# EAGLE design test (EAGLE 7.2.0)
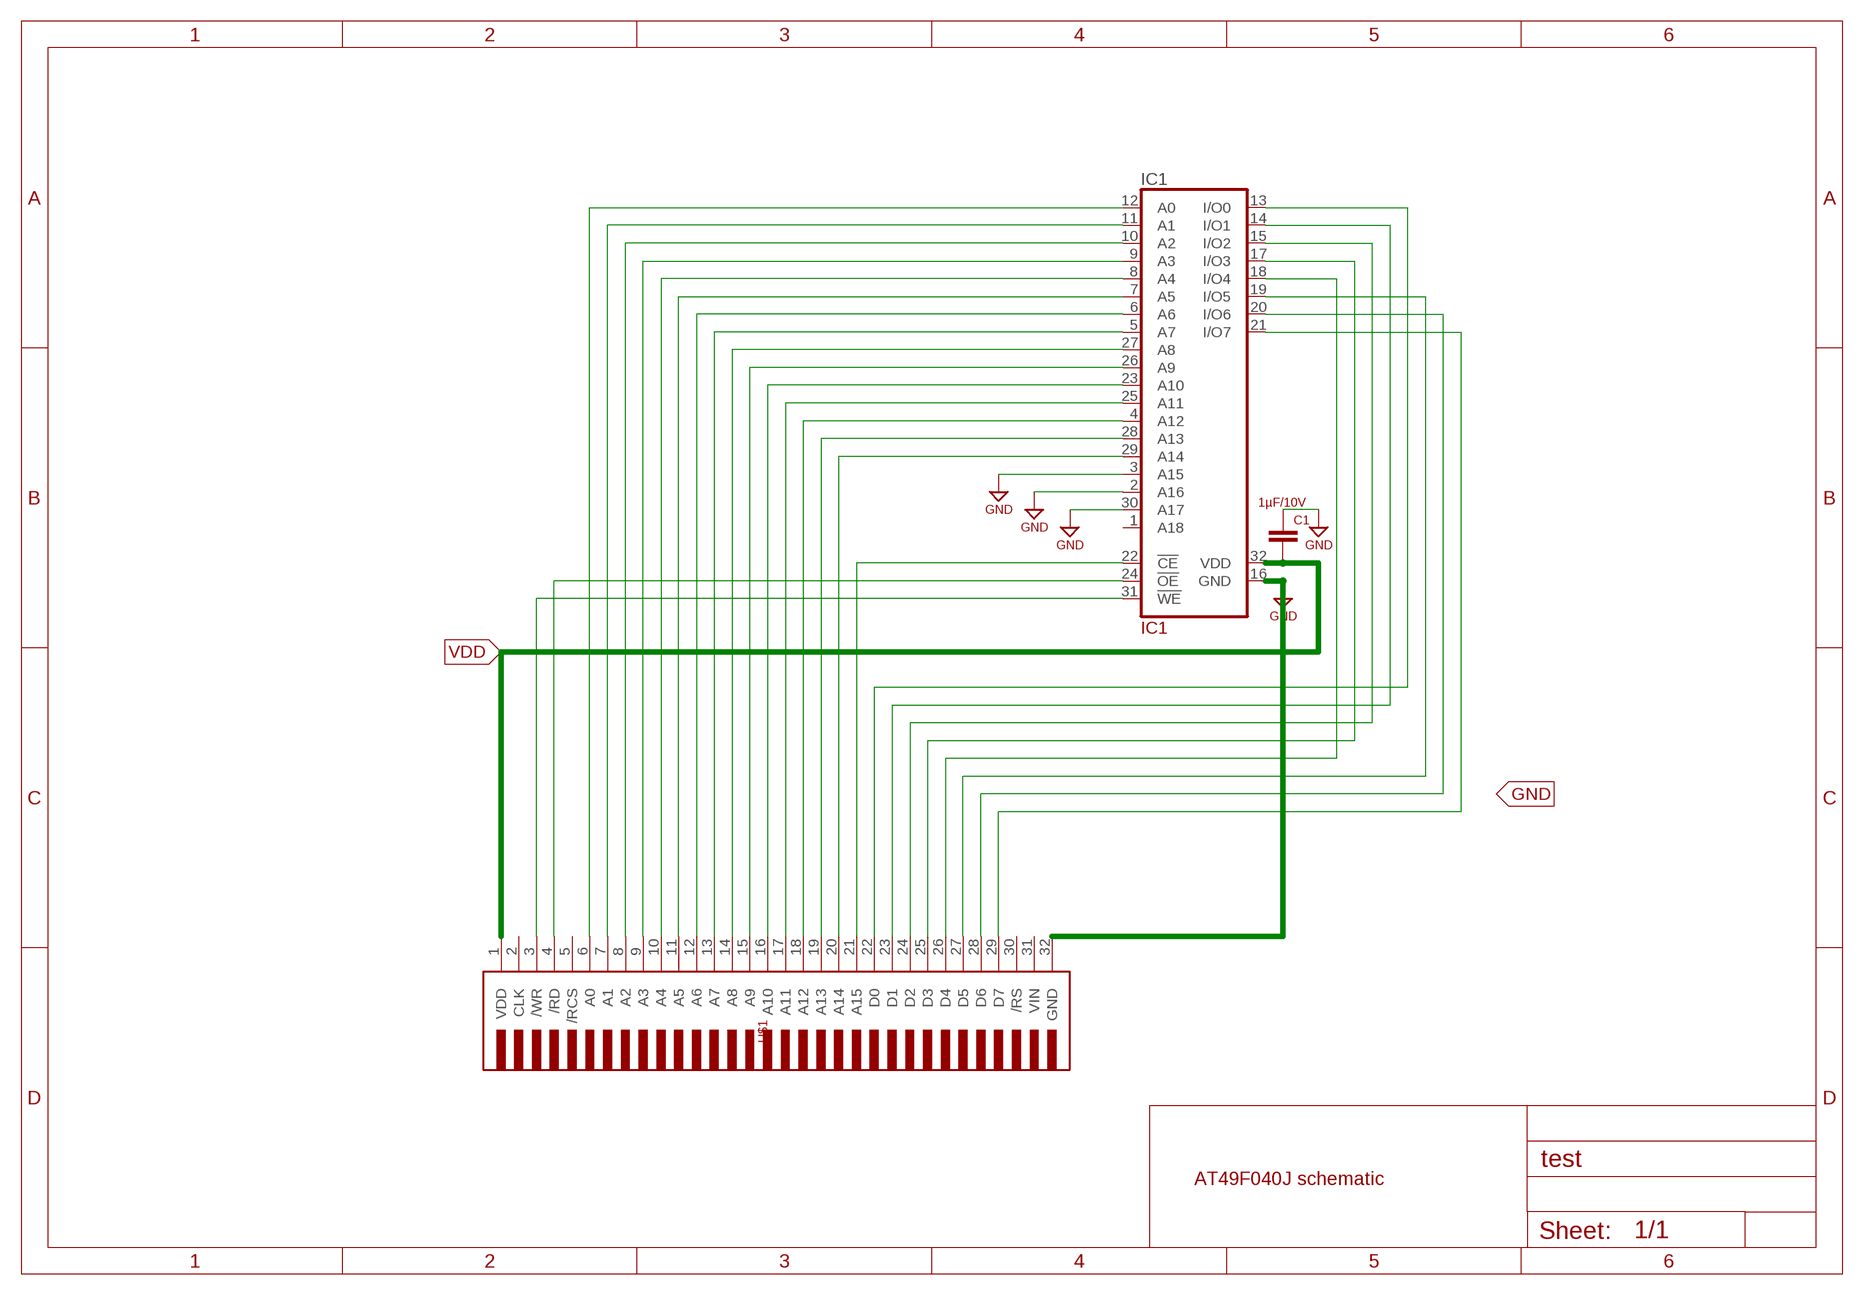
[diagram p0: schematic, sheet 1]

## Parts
C1  1µF/10V  C-EUC0603  [C0603]
IC1  IC1  AT49F040J  [PLCC32R]
U$1  GBCART-FULL  [GBCART]

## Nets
3: IC1.31(!WE) U$1.3(/WR)
4: IC1.24(!OE) U$1.4(/RD)
6: IC1.12(A0) U$1.6(A0)
7: IC1.11(A1) U$1.7(A1)
8: IC1.10(A2) U$1.8(A2)
9: IC1.9(A3) U$1.9(A3)
10: IC1.8(A4) U$1.10(A4)
11: IC1.7(A5) U$1.11(A5)
12: IC1.6(A6) U$1.12(A6)
13: IC1.5(A7) U$1.13(A7)
14: IC1.27(A8) U$1.14(A8)
15: IC1.26(A9) U$1.15(A9)
16: IC1.23(A10) U$1.16(A10)
17: IC1.25(A11) U$1.17(A11)
18: IC1.4(A12) U$1.18(A12)
19: IC1.28(A13) U$1.19(A13)
20: IC1.29(A14) U$1.20(A14)
21: IC1.22(!CE) U$1.21(A15)
22: IC1.13(I/O0) U$1.22(D0)
23: IC1.14(I/O1) U$1.23(D1)
24: IC1.15(I/O2) U$1.24(D2)
25: IC1.17(I/O3) U$1.25(D3)
26: IC1.18(I/O4) U$1.26(D4)
27: IC1.19(I/O5) U$1.27(D5)
28: IC1.20(I/O6) U$1.28(D6)
29: IC1.21(I/O7) U$1.29(D7)
GND: C1.1 IC1.2(A16) IC1.3(A15) IC1.16(GND) IC1.30(A17) U$1.32(GND)
VDD: C1.2 IC1.32(VDD) U$1.1(VDD)
Unconnected: IC1.1(A18) U$1.2(CLK) U$1.5(/RCS) U$1.30(/RS) U$1.31(VIN)

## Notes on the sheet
- AT49F040J schematic

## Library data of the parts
C1 = resistor:C-EU: CAPACITOR, European symbol
IC1 = gameboy:AT49F040J: 4-Megabit FLASH MEMORY (512 K x 8 bit) 5 V-only
U$1 = gameboy_1:GBCART

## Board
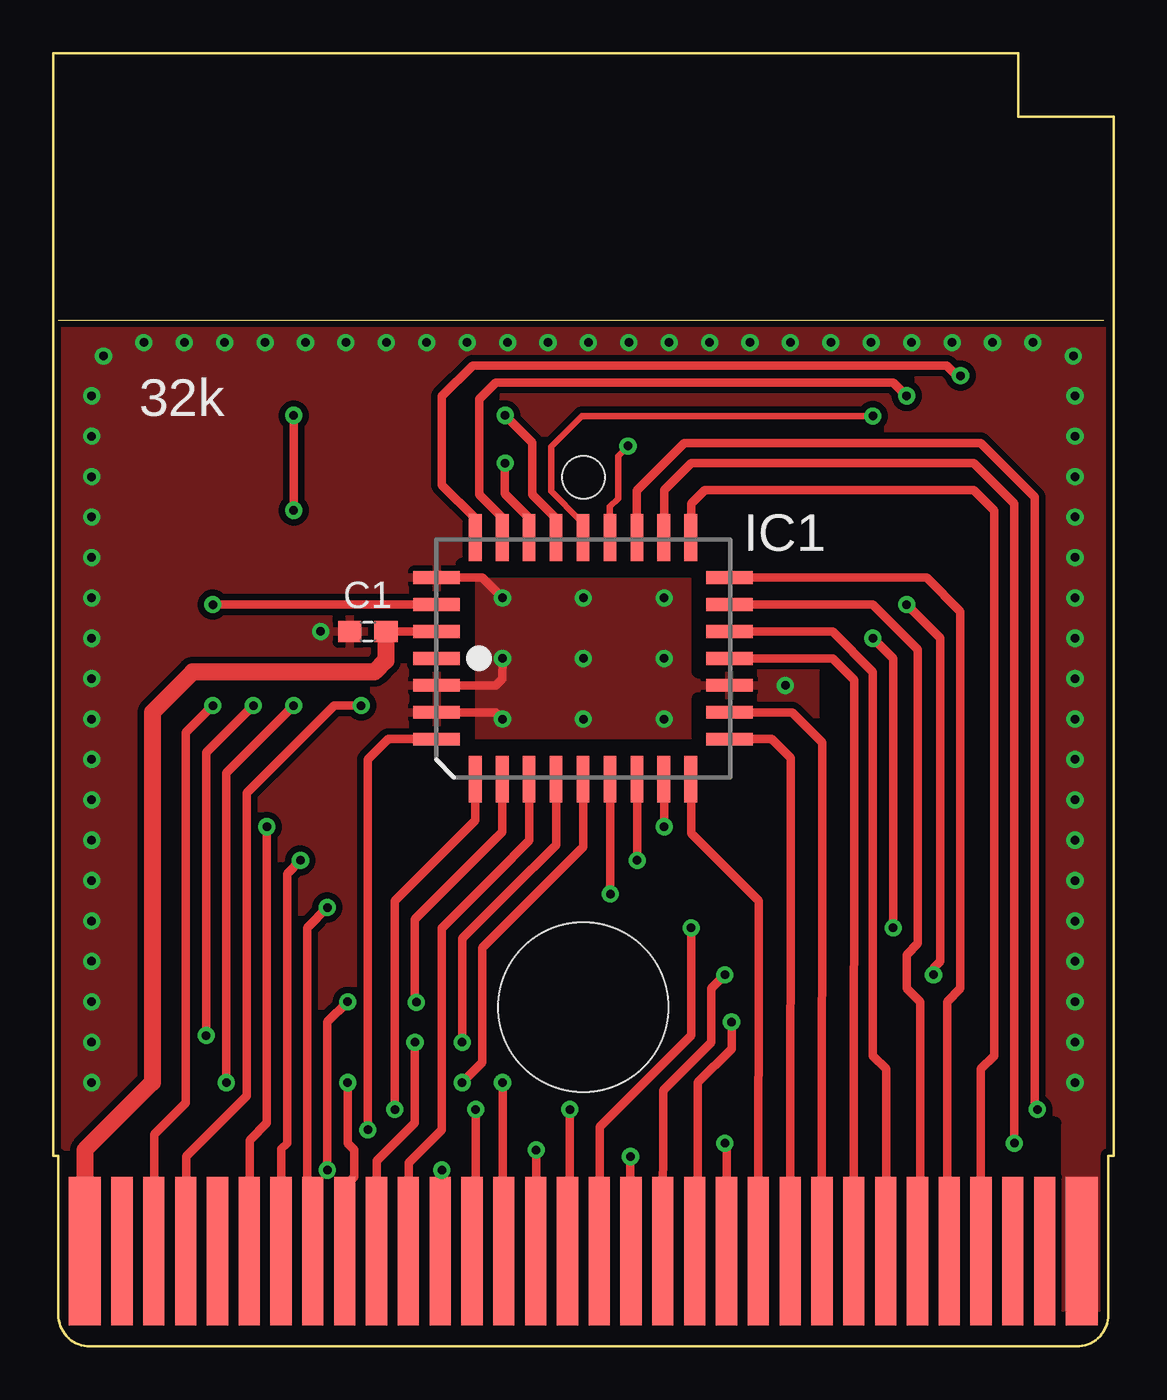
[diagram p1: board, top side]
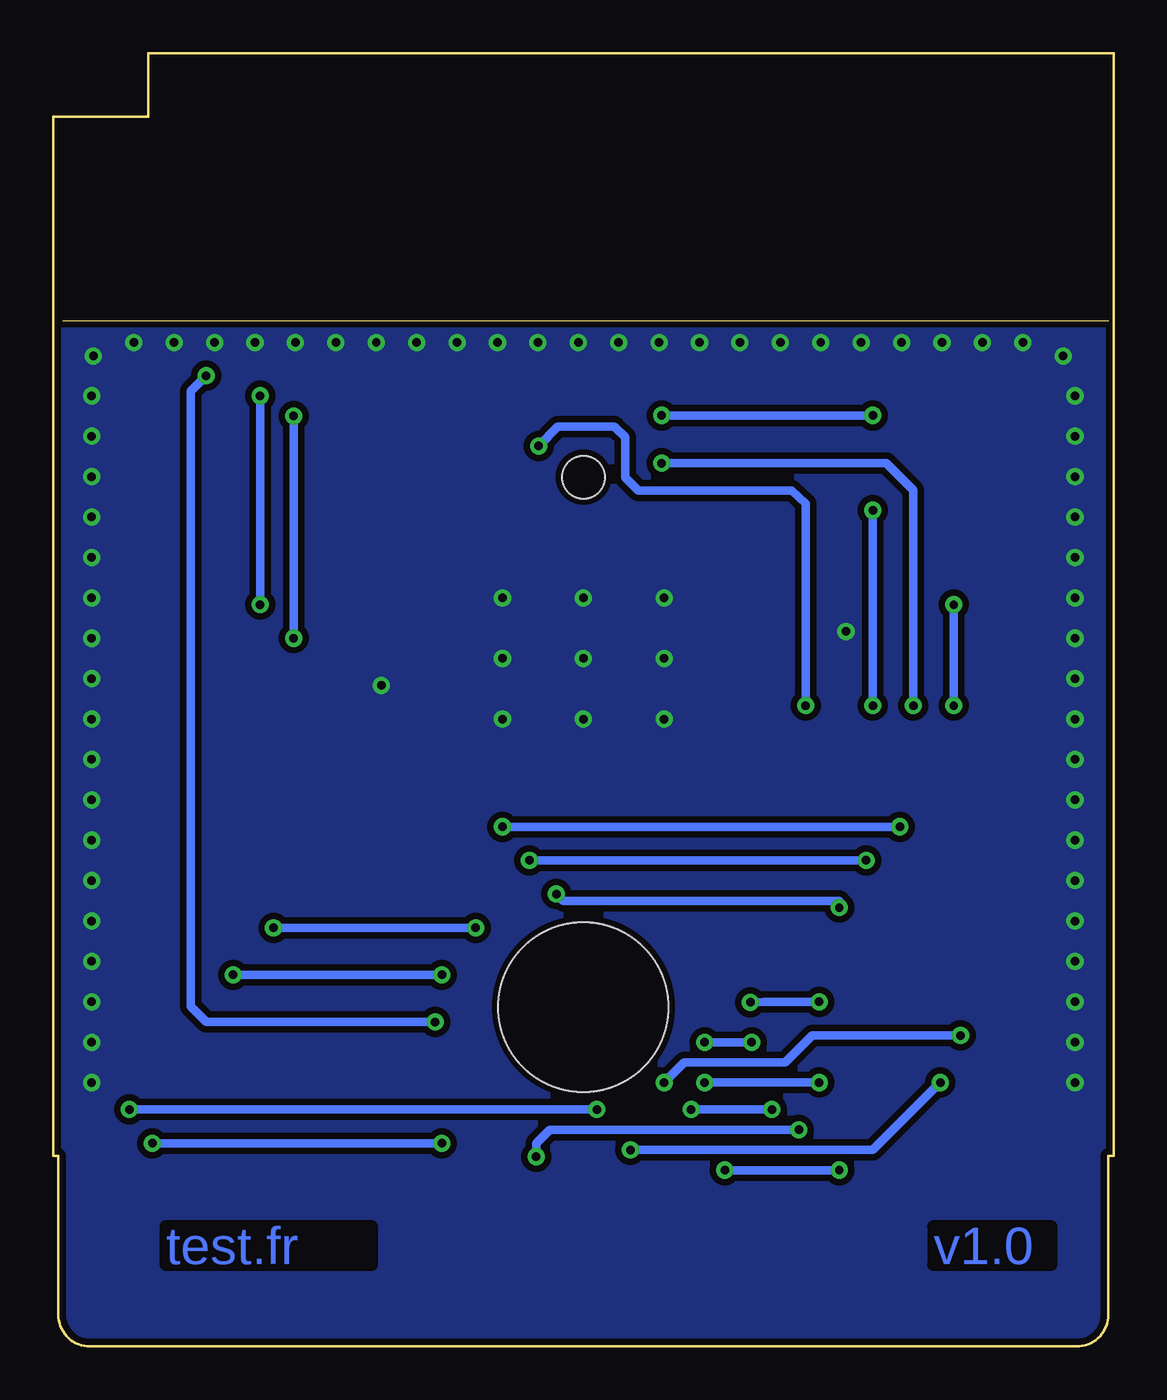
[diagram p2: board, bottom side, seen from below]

Size 50 x 61 mm. Coordinates in mm from the lower left corner, seen from the top.
Outline: 49.53,48.38 0.23,48.38
Copper layers (1*16): Top 0.035mm / dielectric 0.73mm / Bottom 0.035mm
Design rules "default *": minimum track width 10mil, minimum drill 15mil, track to track 8mil, track to pad 8mil, pad to pad 8mil, via to via 8mil, smd to smd 4mil, copper to edge 10mil, drill to drill 8mil, minimum pad ring 10mil, minimum via ring 8mil, stop-mask expansion 4mil, vias tented up to drill 0mil, thermal gap 10mil
tRestrict: area 36.4,7.7 to 37.4,31.8; area 44,7.7 to 45,13.4; area 45,7.4 to 47.2,10.5; area 19.3,28 to 19.6,36.9; area 19.3,36.6 to 30.7,36.9; area 19.3,28 to 31,28.3; area 30.4,31.8 to 30.7,36.6; area 30.4,28 to 30.7,30.5; area 47.2,0.7 to 49.1,1.3

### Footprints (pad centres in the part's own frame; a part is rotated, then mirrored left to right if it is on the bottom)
C0603 = smd 1.1 x 1: 1 -0.85,0; 2 0.85,0
PLCC32R = smd 0.6 x 2.2: 1 0,6.9; 2 -1.27,6.9; 3 -2.54,6.9; 4 -3.81,6.9; 14 -3.81,-6.9; 15 -2.54,-6.9; 16 -1.27,-6.9; 17 0,-6.9; 18 1.27,-6.9; 19 2.54,-6.9; 20 3.81,-6.9; 30 3.81,6.9; 31 2.54,6.9; 32 1.27,6.9 | smd 2.2 x 0.6: 5 -5.7,5.08; 6 -5.7,3.81; 7 -5.7,2.54; 8 -5.7,1.27; 9 -5.7,0; 10 -5.7,-1.27; 11 -5.7,-2.54; 12 -5.7,-3.81; 13 -5.7,-5.08; 21 5.7,-5.08; 22 5.7,-3.81; 23 5.7,-2.54; 24 5.7,-1.27; 25 5.7,0; 26 5.7,1.27; 27 5.7,2.54; 28 5.7,3.81; 29 5.7,5.08
GBCART = smd 1.5 x 7: 1 -23.5,-24.71; 32 23.5,-24.71 | smd 1 x 7: 2 -21.75,-24.71; 3 -20.25,-24.71; 4 -18.75,-24.71; 5 -17.25,-24.71; 6 -15.75,-24.71; 7 -14.25,-24.71; 8 -12.75,-24.71; 9 -11.25,-24.71; 10 -9.75,-24.71; 11 -8.25,-24.71; 12 -6.75,-24.71; 13 -5.25,-24.71; 14 -3.75,-24.71; 15 -2.25,-24.71; 16 -0.75,-24.71; 17 0.75,-24.71; 18 2.25,-24.71; 19 3.75,-24.71; 20 5.25,-24.71; 21 6.75,-24.71; 22 8.25,-24.71; 23 9.75,-24.71; 24 11.25,-24.71; 25 12.75,-24.71; 26 14.25,-24.71; 27 15.75,-24.71; 28 17.25,-24.71; 29 18.75,-24.71; 30 20.25,-24.71; 31 21.75,-24.71 | hole 8: 0,-13.21 | hole 2: 0,11.79

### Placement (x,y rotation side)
C1  14.84,33.72 0 top
IC1  24.98,32.45 90 top
U$1  25,29.21 0 top

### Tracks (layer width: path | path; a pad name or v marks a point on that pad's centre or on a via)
3  (via drill 0.4 pad 0.41)
  Top 0.406: U$1.3 4.77,10 6.27,11.49 6.27,28.96 v7.54,30.23 | v7.54,34.99 IC1.31
  Bottom 0.406: v7.54,30.23 v7.54,34.99
4  (via drill 0.4 pad 0.41)
  Top 0.305: IC1.24 26.25,39.6 26.63,39.98 26.63,42 v27.11,42.47
  Top 0.406: U$1.4 6.27,8.96 9.12,11.81 9.12,26.1 13.25,30.23 v14.52,30.23 | 26.27,38.16 IC1.24
  Bottom 0.406: v14.52,30.23 14.52,39.75 15.18,40.37 22.42,40.37 23.04,40.98 23.04,42.88 23.54,43.38 26.2,43.38 v27.11,42.47
6  (via drill 0.4 pad 0.41)
  Top 0.406: U$1.6 9.27,9.73 10.08,10.54 v10.08,24.51 | v28.81,24.51 28.81,26.73 IC1.12
  Bottom 0.406: v10.08,24.51 v28.81,24.51
7  (via drill 0.4 pad 0.41)
  Top 0.406: U$1.7 10.77,9.33 11.03,9.59 11.03,22.29 v11.66,22.92 | v27.54,22.92 27.54,26.73 IC1.11
  Bottom 0.406: v11.66,22.92 v27.54,22.92
8  (via drill 0.4 pad 0.41)
  Top 0.406: v26.27,21.34 26.27,26.73 IC1.10 | v12.93,20.7 11.98,19.75 11.98,7.37 12.3,7.05 12.3,4.4 U$1.8
  Bottom 0.406: v26.27,21.34 25.95,21.02 12.93,21.02 v12.93,20.7
9  (via drill 0.4 pad 0.41)
  Top 0.406: 13.77,12.33 v13.89,12.45 13.89,9.59 14.21,9.27 14.21,8 13.77,7.57 U$1.9 | v19.29,12.45 20.24,13.4 20.24,18.8 25,23.56 25,26.73 IC1.9
  Bottom 0.406: v13.89,12.45 v19.29,12.45
10  (via drill 0.4 pad 0.41)
  Top 0.406: IC1.8 23.71,23.66 21.52,21.49 19.29,19.25 v19.29,14.35 | U$1.10 15.27,8.75 17.06,10.54 v17.06,14.35
  Bottom 0.406: v17.06,14.35 v19.29,14.35
11
  Top 0.406: IC1.7 22.45,23.86 20.86,22.26 18.35,19.75 18.33,19.75 18.33,10.22 16.77,8.66 U$1.11
12  (via drill 0.4 pad 0.41)
  Top 0.406: IC1.6 21.18,24.26 17.06,20.14 17.06,16.26 17.04,16.23 v17.13,16.23 | U$1.12 18.27,7.94 v18.33,8.32 | v12.93,8.32 12.93,15.3 v13.89,16.26
  Bottom 0.406: v18.33,8.32 v12.93,8.32 | v13.89,16.26 16.47,16.26 v17.13,16.23
13  (via drill 0.4 pad 0.41)
  Top 0.406: v19.92,11.18 19.92,4.52 U$1.13 | IC1.5 19.91,24.81 16.11,21.02 v16.11,11.18
  Bottom 0.406: v16.11,11.18 v19.92,11.18
14  (via drill 0.4 pad 0.41)
  Top 0.406: v7.22,14.67 7.22,28 v9.44,30.23 | 22.46,38.16 IC1.27 22.45,39.07 21.29,40.23 21.29,41.63 v21.31,41.66 | U$1.14 21.19,4.45 v21.19,12.45
  Bottom 0.406: v7.22,14.67 14.21,14.67 15.47,13.4 20.24,13.4 v21.19,12.45 | v9.44,30.23 9.44,40.39 10.71,41.66 v21.31,41.66
15  (via drill 0.4 pad 0.41)
  Top 0.406: U$1.15 22.77,8.96 v22.78,9.27 | v8.17,12.45 8.17,27.05 v11.35,30.23 | v11.35,39.43 v11.35,43.91 | IC1.26 23.72,39.04 22.59,40.18 22.59,42.64 v21.31,43.91
  Bottom 0.406: v22.78,9.27 11.35,9.27 v8.17,12.45 | v11.35,30.23 v11.35,39.43 | v11.35,43.91 v21.31,43.91
16  (via drill 0.4 pad 0.41)
  Top 0.406: IC1.23 27.52,40.37 29.76,42.61 43.73,42.61 46.27,40.07 46.27,11.3 v46.4,11.18 | v24.36,11.18 24.36,4.46 U$1.16
  Bottom 0.406: v46.4,11.18 v24.36,11.18
17  (via drill 0.4 pad 0.41)
  Top 0.305: v38.65,43.88 24.93,43.88 23.48,42.43 23.48,40.33 24.84,38.98 25,38.97
  Top 0.406: v30.08,19.75 30.08,14.67 25.77,10.36 U$1.17 | v39.6,19.75 39.6,32.45 v38.65,33.4 | IC1.25 25,38.16 25,38.97 | v38.65,43.88
  Bottom 0.406: v30.08,19.75 v39.6,19.75 | v38.65,33.4 v38.65,43.88
18  (via drill 0.4 pad 0.41)
  Top 0.406: IC1.4 15.79,28.64 14.84,27.69 v14.84,10.22 | v27.22,8.95 27.22,4.41 U$1.18
  Bottom 0.406: v14.84,10.22 26.59,10.22 27.22,9.59 v27.22,8.95
19  (via drill 0.4 pad 0.41)
  Top 0.406: U$1.19 28.77,12.09 31.03,14.35 31.03,16.89 v31.67,17.53 | 21.19,38.16 IC1.28 21.13,38.19 21.13,39.13 20.09,40.18 20.09,44.68 20.88,45.47 39.6,45.47 v40.24,44.83 | v40.24,34.99 41.83,33.4 41.83,18.16 41.51,17.84 v41.51,17.53
  Bottom 0.406: v31.67,17.53 v41.51,17.53 | v40.24,34.99 v40.24,44.83
20  (via drill 0.4 pad 0.41)
  Top 0.406: U$1.20 30.4,4.49 30.4,12.45 31.98,14.03 v31.98,15.3 | v42.78,45.78 42.61,45.78 42.13,46.26 19.78,46.26 18.34,44.81 18.34,40.63 19.91,39.06 IC1.29
  Bottom 0.406: v31.98,15.3 42.78,15.3 43.52,16.04 43.52,45.05 v42.78,45.78
21  (via drill 0.4 pad 0.41)
  Top 0.406: U$1.21 31.77,9.49 v31.67,9.59 | v45.32,9.59 45.32,39.75 43.41,41.66 30.08,41.66 28.81,40.39 28.81,38.16 IC1.22
  Bottom 0.406: v31.67,9.59 v45.32,9.59
22
  Top 0.406: U$1.22 33.27,21 30.08,24.19 30.08,26.73 IC1.13
23
  Top 0.406: U$1.23 34.77,27.76 33.89,28.64 IC1.14
24
  Top 0.406: U$1.24 36.27,28.48 34.84,29.91 IC1.15
25
  Top 0.406: U$1.25 37.77,31.43 36.75,32.45 IC1.17
26
  Top 0.406: IC1.18 36.75,33.72 38.65,31.81 38.65,13.72 39.29,13.08 39.29,4.38 U$1.26
27
  Top 0.406: IC1.19 38.65,34.99 40.77,32.87 40.77,19.01 40.24,18.48 40.24,16.89 40.88,16.26 40.88,4.47 U$1.27
28
  Top 0.406: U$1.28 42.14,4.49 42.14,16.26 42.78,16.89 42.78,34.67 41.19,36.26 IC1.20
29
  Top 0.406: IC1.21 30.08,38.16 30.08,39.75 30.71,40.39 43.41,40.39 44.37,39.43 44.37,13.72 43.73,13.08 43.73,4.4 U$1.29
GND  (via drill 0.4)
  Top 0.406: IC1.2 20.88,31.18 21.18,31.48 v21.19,32.45 | IC1.3 20.87,29.91 v21.19,29.59 | IC1.30 20.24,36.26 v21.19,35.31
  other vias: 2.38,46.71 4.28,47.35 6.19,47.35 8.09,47.35 10,47.35 11.9,47.35 13.81,47.35 15.71,47.35 17.62,47.35 19.52,47.35 21.43,47.35 23.33,47.35 25.24,47.35 29.05,47.35 30.95,47.35 32.86,47.35 34.76,47.35 36.67,47.35 38.57,47.35 40.48,47.35 42.38,47.35 44.29,47.35 46.19,47.35 48.18,33.4 48.18,31.5 48.18,29.59 48.18,27.69 48.18,25.78 48.18,23.88 48.18,21.97 48.18,20.07 48.18,18.16 48.18,16.26 48.18,14.35 48.18,12.45 1.82,33.4 1.82,31.5 1.82,29.59 1.82,27.69 1.82,25.78 1.82,23.88 1.82,21.97 1.82,20.07 1.82,18.16 1.82,16.26 1.82,14.35 1.82,12.45 25,35.31 28.81,35.31 28.81,32.45 28.81,29.59 25,29.59 25,32.45 27.14,47.35 1.82,35.31 1.82,37.21 48.18,37.21 48.18,35.31 48.1,46.71 1.82,39.12 1.82,41.02 1.82,42.93 1.82,44.83 48.18,39.12 48.18,41.02 48.18,42.93 48.18,44.83 34.52,31.18 12.62,33.72
  pour Top (isolate 0.305): -0.27,49.91 50.27,49.91 50.27,-0.02 -0.27,-0.02
  pour Bottom (isolate 0.305): -0.27,49.91 50.27,49.91 50.27,-0.02 -0.27,-0.02
VDD
  Top 0.406: C1.2 IC1.32 | 1.5,4.43 U$1.1
  Top 0.813: C1.2 15.69,32.35 15.16,31.81 6.58,31.81 4.68,29.91 4.68,12.45 1.5,9.27 1.5,4.43

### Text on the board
Bottom: v1.0 | test.fr
tPlace: 32k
